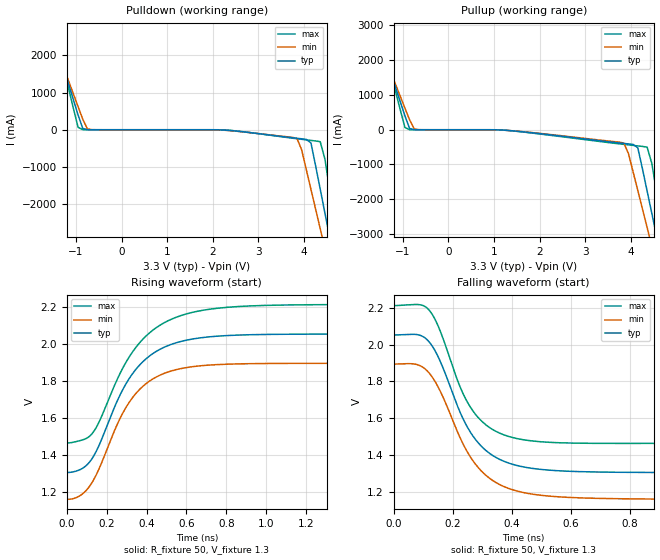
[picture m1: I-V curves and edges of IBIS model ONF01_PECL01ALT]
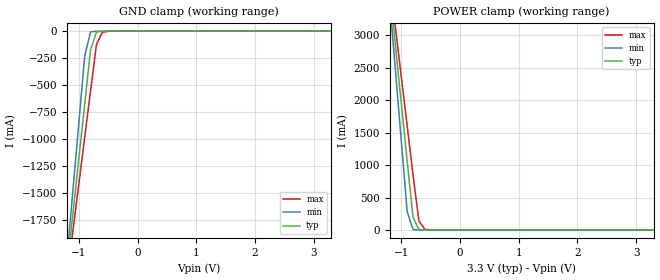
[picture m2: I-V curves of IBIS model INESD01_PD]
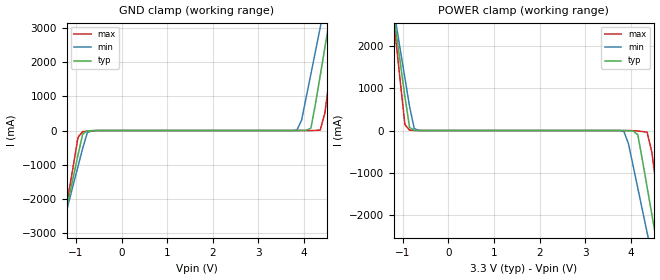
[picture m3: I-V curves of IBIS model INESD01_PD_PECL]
|   This file is an IBIS representation of the   |
|   Integrated Circuit Systems, Inc.   |
|   ICS85304-01   |
|   Low Skew 1 to 5 LVPECL 3.3V Clock Buffer   |
[IBIS Ver]   4.1
[File name]   85304_01_3v3.ibs
[File Rev]   0.0
[Date]   11 Dec 2008 | Last modified
|   05 Jul 2001 | Generated
[Source]   Originated at Integrated Devices Technology, Inc.
[Disclaimer]
IDT hereby grants the user of this IBIS model a non-exclusive,
nontransferable license to use this IBIS model under the following terms.
Before using this IBIS model, the user should read this license.
If the user does not accept these terms,  the IBIS model should be
returned to IDT within 30 days.
   The user is granted this license only to use the IBIS model and
is not granted rights to sell, load, rent, lease or license the IBIS
model in whole or in part, or in modified form to anyone other than
user. User may modify the IBIS model to suit its specific
applications but rights to derivative works and such modifications
shall belong to IDT.
   This IBIS model is provided on an "AS IS" basis and IDT makes
absolutely no warranty with respect to the information contained
herein. IDT DISCLAIMS AND CUSTOMER WAIVES ALL WARRANTIES, EXPRESS
OR IMPLIED, INCLUDING WARRANTIES OF MERCHANTABILITY OR FITNESS FOR
A PARTICULAR PURPOSE. The entire risk as to quality and performance
is with the Customer. ACCORDINGLY, IN NO EVENT SHALL THE COMPANY BE
LIABLE FOR ANY DAMAGES, WHETHER IN CONTRACT OR TORT,INCLUDING ANY
LOST PROFITS OR OTHER INCIDENTAL, CONSEQUENTIAL, EXEMPLARY, OR
PUNITIVE DAMAGES ARISING OUT OF THE USE OR APPLICATION OF THE IBIS
model provided in this package. Further, IDT reserves the right to
make changes without notice to any product herein to improve
reliability, function, or design. IDT does not convey any license
under patent rights or any other intellectual property rights,
including those of third parties.
   IDT is not obligated to provide maintenance or support
for the licensed IBIS model.
[Copyright]   Copyright 2001 by Integrated Device Technology, Inc.
[Component]   85304AG_01
[Manufacturer] Integrated Devices Technology, Inc.
[Package]
|TSSOP 20 Lead
|   typ   min   max
R_pkg   51.85m   41.1m   62.6m
L_pkg   1.568nH   0.734nH   2.401nH
C_pkg   0.221pF   0.068pF   0.373pF
[Pin]   signal_name   model_name   R_pin   L_pin   C_pin
1   Q0   ONF01_PECL01ALT   62.6m   2.401n   0.373p
2   nQ0   ONF01_PECL01ALT   57.23m   1.985n   0.297p
3   Q1   ONF01_PECL01ALT   51.85m   1.568n   0.221p
4   nQ1   ONF01_PECL01ALT   46.78m   1.151n   0.145p
5   Q2   ONF01_PECL01ALT   41.1m   0.734n   0.068p
6   nQ2   ONF01_PECL01ALT   41.1m   0.734n   0.068p
7   Q3   ONF01_PECL01ALT   46.78m   1.151n   0.145p
8   nQ3   ONF01_PECL01ALT   51.85m   1.568n   0.221p
9   Q4   ONF01_PECL01ALT   57.23m   1.985n   0.297p
10   nQ4   ONF01_PECL01ALT   62.6m   2.401n   0.373p
11   VCC   POWER   62.6m   2.401n   0.373p
12   CLK_SEL   INESD01_PD   57.23m   1.985n   0.297p
13   CLK0   INESD01_PD_PECL   51.85m   1.568n   0.221p
14   nCLK0   INESD01_PU_PECL   46.78m   1.151n   0.145p
15   VEE   GND   41.1m   0.734n   0.068p
16   CLK1   INESD01_PD_PECL   41.1m   0.734n   0.068p
17   nCLK1   INESD01_PU_PECL   46.78m   1.151n   0.145p
18   VCC   POWER   51.85m   1.568n   0.221p
19   CLK_EN   INESD01_PU   57.23m   1.985n   0.297p
20   VCC   POWER   62.6m   2.401n   0.373p
[Diff Pin]  inv_pin  vdiff tdelay_typ tdelay_min  tdelay_max
1   2   NA   0   0   0
3   4   NA   0   0   0
5   6   NA   0   0   0
7   8   NA   0   0   0
9   10   NA   0   0   0
| Models and submodels in the file (5): ONF01_PECL01ALT (Output_ECL), INESD01_PD (Input), INESD01_PD_PECL (Input), INESD01_PU_PECL (Input), INESD01_PU (Input)
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[Model]   ONF01_PECL01ALT
Model_type  Output_ECL
Polarity   Non-Inverting
Vmeas = 1.636
Rref = 50
Cref = 0
Vref = 1.3
|Variable  typ   min   max
C_comp   2p   1.5p   2.5p
[Voltage Range]   3.3   3.135   3.465
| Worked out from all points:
|   rising waveform, R_fixture 50, V_fixture 1.3: 20-80 % time 218ps typ, 206ps min, 242ps max; typ from 1.31 V to 2.05 V
|   falling waveform, R_fixture 50, V_fixture 1.3: 20-80 % time 134ps typ, 143ps min, 120ps max; typ from 2.05 V to 1.31 V
| Open source, no load
|  Voltage   I(typ)   I(min)   I(max)
[Pullup]
-3.3V     9.786A     8.45A      12.03A
-1.667V   3.247A     2.997A     3.691A
-1.565V   2.839A     2.657A     3.17A
-952.6mV  398mA      622.1mA    64.71mA
-850.5mV  36.63mA    284.2mA    1.532mA
-646.4mV  229.3uA    1.611mA    19.07uA
3.844V    -394.4mA   -383.6mA   -421.3mA
4.151V    -517.8mA   -1.749A    -465.4mA
4.355V    -1.764A    -2.812A    -500.3mA
4.559V    -3.036A    -3.875A    -1.773A
4.763V    -4.308A    -4.937A    -3.393A
6.6V      -15.79A    -14.52A    -18.03A
[Pulldown]
-3.3V     9.786A     8.45A      12.03A
-1.565V   2.839A     2.657A     3.17A
-1.463V   2.432A     2.317A     2.65A
-952.6mV  398mA      622.1mA    64.71mA
-850.5mV  36.63mA    284.2mA    1.532mA
-646.4mV  229.3uA    1.611mA    19.07uA
3.844V    -229.1mA   -232.1mA   -241.8mA
4.151V    -352.7mA   -1.598A    -286.7mA
4.355V    -1.599A    -2.66A     -322.1mA
4.559V    -2.871A    -3.722A    -1.595A
4.763V    -4.144A    -4.785A    -3.217A
6.6V      -15.69A    -14.41A    -17.97A
[Ramp]
|   typ   min   max
dV/dt_r   0.45V/0.37ns   0.45V/0.405ns   0.45V/0.27ns
dV/dt_f   0.45V/0.37ns   0.45V/0.405ns   0.45V/0.27ns
R_load =   50.0000
[Rising Waveform]
R_fixture = 50
V_fixture = 1.3   | VCC_typ - 2V
V_fixture_max = 1.465   | VCC_max - 2V
V_fixture_min = 1.135   | VCC_min - 2V
C_fixture = 0.0p
| Time   typ   min   max
0s        1.306V     1.161V     1.465V
70ps      1.323V     1.183V     1.479V
128ps     1.383V     1.254V     1.517V
258ps     1.703V     1.577V     1.819V
316ps     1.817V     1.689V     1.934V
398ps     1.919V     1.785V     2.042V
504ps     1.988V     1.846V     2.121V
658ps     2.03V      1.879V     2.175V
875ps     2.047V     1.891V     2.201V
2ns       2.052V     1.894V     2.211V
[Falling Waveform]
R_fixture = 50
V_fixture = 1.3   | VCC_typ - 2V
V_fixture_max = 1.465   | VCC_max - 2V
V_fixture_min = 1.135   | VCC_min - 2V
C_fixture = 0.0p
0s        2.052V     1.894V     2.211V
76ps      2.055V     1.893V     2.217V
118ps     2.018V     1.85V      2.19V
150ps     1.936V     1.772V     2.103V
222ps     1.644V     1.505V     1.782V
264ps     1.514V     1.38V      1.65V
326ps     1.409V     1.274V     1.549V
410ps     1.348V     1.21V      1.493V
708ps     1.309V     1.166V     1.465V
2ns       1.306V     1.161V     1.465V
[Model]   INESD01_PD
Model_type   Input
Polarity   Non-Inverting
Vinl = 0.80V
Vinh = 2.0V
|   typ   min   max
C_comp   2pF   1.5pF   2.5pF
|   typ   min   max
[Voltage range]  3.3V   3.15V   3.45V
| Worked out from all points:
|   GND clamp passes 1 mA (typ) near -0.55 V on its own axis
|   POWER clamp passes 1 mA (typ) near -0.60 V on its own axis
[GND_clamp]
|Voltage I(typ)   I(min)   I(max)
-3.3V     -12.83A    -15.14A    -11.37A
-1.2V     -2.195A    -2.092A    -2.281A
-1.1V     -1.689A    -1.472A    -1.849A
-900mV    -678.5mA   -232.6mA   -984.8mA
-800mV    -173.9mA   -7.175mA   -553.2mA
-700mV    -9.696mA   -1.052mA   -126mA
-600mV    -1.629mA   -178uA     -11.07mA
-300mV    -10.53uA   -5.678uA   -86.08uA
3.3V      71.13uA    62.11uA    77.58uA
[POWER_clamp]
|Voltage   I(typ)   I(min)   I(max)
-3.3V     22.38A     26.45A     19.82A
-1.2V     3.723A     3.545A     3.874A
-1.1V     2.836A     2.457A     3.116A
-1V       1.949A     1.369A     2.358A
-900mV    1.063A     281.1mA    1.601A
-800mV    191.6mA    5.074mA    844mA
-700mV    8.104mA    204.3uA    138.4mA
-600mV    678.1uA    79.74uA    10.7mA
-400mV    87.44uA    69.65uA    413.2uA
3.3V      -3.041nA   -425fA     -919.9nA
[Model]   INESD01_PD_PECL
Model_type  Input
Polarity   Non-Inverting
Vinl = 0.8V
Vinh = 2.0V
|   typ   min   max
C_comp   2pF   1.5pF   2.5pF
|   typ   min   max
[Voltage range]  3.3V   3.15V   3.45V
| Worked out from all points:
|   GND clamp passes 1 mA (typ) near -0.55 V on its own axis
|   POWER clamp passes 1 mA (typ) near -0.66 V on its own axis
[GND_clamp]
|Voltage   I(typ)   I(min)   I(max)
-2.586V   -10.86A    -9.487A    -13.15A
-1.361V   -3.24A     -3.145A    -3.432A
-1.259V   -2.606A    -2.617A    -2.622A
-952.6mV  -705.3mA   -1.038A    -192.4mA
-850.5mV  -99.9mA    -513.5mA   -31.23mA
-646.4mV  -3.788mA   -3.549mA   -8.297mA
3.844V    129.1uA    13.13mA    71.12uA
4.151V    73.33mA    1.652A     864.7uA
4.355V    1.607A     3.003A     15.44mA
4.559V    3.233A     4.356A     1.553A
4.763V    4.861A     5.711A     3.635A
5.375V    9.757A     9.783A     9.893A
[POWER_clamp]
|Voltage   I(typ)   I(min)   I(max)
-2.177V   10.57A     9.364A     12.62A
-1.157V   2.42A      2.586A     2.194A
-952.6mV  795.8mA    1.237A     137.8mA
-850.5mV  73.33mA    563.2mA    8.145mA
-646.4mV  535.8uA    2.004mA    431.2uA
3.844V    -826.3uA   -18.14mA   -47.07uA
4.151V    -99.9mA    -1.362A    -11.82mA
4.355V    -1.338A    -2.415A    -41.71mA
4.559V    -2.606A    -3.47A     -1.312A
4.661V    -3.24A     -3.998A    -2.123A
4.763V    -3.875A    -4.526A    -2.933A
5.579V    -8.954A    -8.756A    -9.414A
